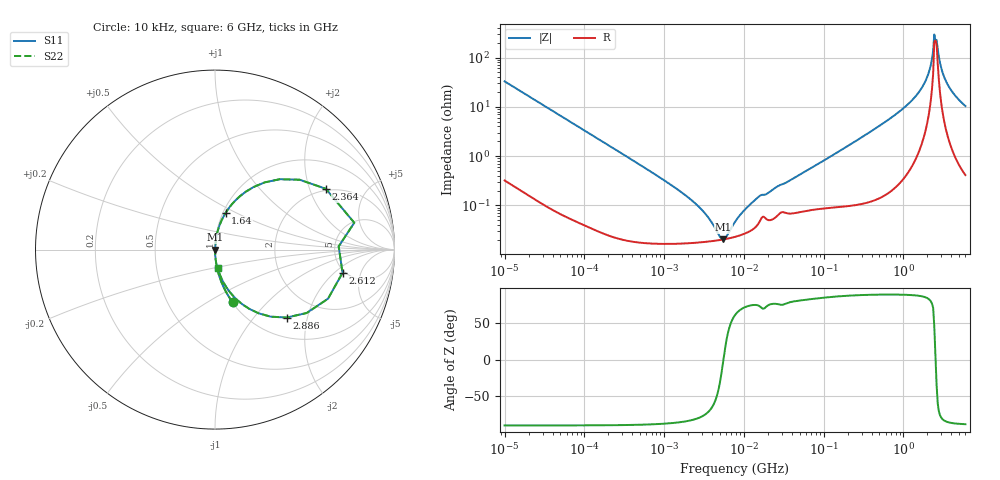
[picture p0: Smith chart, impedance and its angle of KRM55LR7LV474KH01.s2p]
!Murata Part Number: KRM55LR7LV474KH01
!These Parameters are Measured in Series Mode Connection
!Data Generated on Jan 08, 2026
!  o--ll--o
!Port1  Port2
!  o------o
!Operation Temp=25[degC], DC Bias Voltage=0[V]
!Freq. Start=10[kHz] Stop=6[GHz] 401[Steps]
# Hz S RI R 50
!Freq.(Hz) S11(Real) S11(Imag) S21(Real) S21(Imag) S12(Real) S12(Imag) S22(Real) S22(Imag)
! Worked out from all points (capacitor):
!   401 points, 10 kHz to 6 GHz, reference 50 ohm
!   read as one part in series: C = 484 nF near 10.69 kHz
!   lowest |Z| = 20.4 mohm at 5.554 MHz (marker M1)
!   series resonance near 5.547 MHz, so ESL is about 1.7 nH
!   S11 on the Smith chart (normalised r, x): 10 kHz: 1.01, -0.66; 1.64 GHz: 1.03, +0.44; 2.364 GHz: 1.93, +2.60; 2.612 GHz: 4.76, -2.57; 2.886 GHz: 1.38, -1.50; 6 GHz: 1.01, -0.21
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10000  0.0996 -0.2947  0.9004 0.2947  0.9004 0.2947  0.0996 -0.2947
27124  0.0157 -0.1197  0.9843 0.1197  0.9843 0.1197  0.0157 -0.1197
92862  0.00169 -0.0357  0.9983 0.0357  0.9983 0.0357  0.00169 -0.0357
862344  0.00018 -0.00378  0.9998 0.00378  0.9998 0.00378  0.00018 -0.00378
2671920  0.000177 -0.000952  0.9998 0.000952  0.9998 0.000952  0.000177 -0.000952
5026732  0.000198 -0.000117  0.9998 0.000117  0.9998 0.000117  0.000198 -0.000117
5554204  0.000204 1.6e-06  0.9998 -1.6e-06  0.9998 -1.6e-06  0.000204 1.6e-06
7745967  0.00023 0.000401  0.9998 -0.000401  0.9998 -0.000401  0.00023 0.000401
1.557502e7  0.000456 0.00145  0.9995 -0.00145  0.9995 -0.00145  0.000456 0.00145
7.193098e7  0.000842 0.00583  0.9992 -0.00583  0.9992 -0.00583  0.000842 0.00583
6.67969e8  0.005 0.0561  0.995 -0.0561  0.995 -0.0561  0.005 0.0561
1.137319e9  0.0167 0.1095  0.9833 -0.1095  0.9833 -0.1095  0.0167 0.1095
1.639765e9  0.0589 0.2042  0.9411 -0.2042  0.9411 -0.2042  0.0589 0.2042
2.001953e9  0.1727 0.3233  0.8273 -0.3233  0.8273 -0.3233  0.1727 0.3233
2.212024e9  0.3602 0.3921  0.6398 -0.3921  0.6398 -0.3921  0.3602 0.3921
2.364181e9  0.6175 0.3388  0.3825 -0.3388  0.3825 -0.3388  0.6175 0.3388
2.526803e9  0.6891 0.018  0.3109 -0.018  0.3109 -0.018  0.6891 0.018
2.612262e9  0.7106 -0.1291  0.2894 0.1291  0.2894 0.1291  0.7106 -0.1291
2.886376e9  0.3989 -0.3787  0.6011 0.3787  0.6011 0.3787  0.3989 -0.3787
3.189254e9  0.1914 -0.3304  0.8086 0.3304  0.8086 0.3304  0.1914 -0.3304
3.523913e9  0.1041 -0.2614  0.8959 0.2614  0.8959 0.2614  0.1041 -0.2614
6e9  0.0146 -0.1016  0.9854 0.1016  0.9854 0.1016  0.0146 -0.1016
